| IBIS file generated by GenIBIS.pl Version 2.11
|   omap3530cbb
[IBIS ver]   4.1
[File name]   omap3530cbb.ibs
[File Rev]   1.0
[Date]   Wed Dec 9, 2009, 14:25:37
[Source]   Data created at Texas Instruments
[Notes]   1) Model checked with IBISCHK4 and contains...
   16 errors relating to DC endpoints. These errors can be waived
   and relate to special modelling of active feedback IOs.
   182 warnings relating to non-monotonic behavior, non-zero
   GND/POWER Clamp values and C_comp max/min values. These
   warnings can be waived.
[Disclaimer] Please be aware that in the absence of a written agreement,
   Texas Instruments (TI) assumes no liability for: 1) the
   accuracy of the IBIS models provided to your company, 2) the
   proper functioning of these IBIS models in your design or for
   any resulting applications, or, 3) infringement of patents,
   copyrights, or intellectual property rights resulting from
   your use of these IBIS models. TI provides IBIS models as a
   service to our customers and therefore reserves the right to
   limit distribution of the IBIS models.
[Copyright]   Property of Texas Instruments Incorporated. Unauthorised
   reproduction and/or distribution is strictly prohibited. This
   product is protected under copyright law and trade secret law
   as an unpublished work. Created 1999,(C) Copyright 1999-2001,
   Texas Instruments Incorporated., All Rights Reserved. These
   commodities are under the U.S. Government distribution license
   control.As such,they are not to be re-exported without the
   prior approval of the U.S. Department of Commerce.
|   Component omap3530cbb
[Component]   omap3530cbb
[Manufacturer]   Texas Instruments.
[Package Model] omap3530cbb
[Package]
|   typ   min   max
R_pkg   0.4048305   2.97780e-002   7.79883e-001
L_pkg   4.2681365E-009 -2.79127e-010  8.81540e-009
C_pkg   1.649116E-012  -6.89568e-013  3.98780e-012
[Pin]   signal_name   model_name
A4   sdrc_a0   Selector8
A6   sdrc_dqs0   Selector1
A7   sdrc_d5   Selector11
A9   sdrc_d7   Selector11
A10   sdrc_dqs2   Selector1
A11   sdrc_d21   Selector11
A16   sdrc_dm1   Selector8
A17   sdrc_dqs1   Selector1
A19   sdrc_d25   Selector11
A20   sdrc_dqs3   Selector1
A25   cam_d5   Selector1
AA3   mcspi2_clk   Selector1
AA4   mcspi1_somi   Selector15
AA8   uart1_tx   Selector1
AA9   uart1_rts   Selector1
AA12   jtag_rtck   Selector6
AA17   jtag_ntrst   Selector27
AA19   jtag_tdo   Selector6
AA25   uart2_tx   Selector23
AA27   dss_data15   Selector24
AA28   dss_data14   Selector24
AB1   mcspi1_cs2   Selector15
AB4   mcspi1_simo   Selector15
AB25   uart2_rts   Selector23
AB26   uart2_cts   Selector23
AB27   dss_data13   Selector24
AC3   mcspi1_cs1   Selector15
AC27   dss_data22   Selector24
AD1   mcbsp4_dr   Selector1
AD27   dss_data11   Selector24
AE1   mcbsp4_clkx   Selector1
AE3   mmc2_dat7   Selector1
AE5   mcbsp3_fsx   Selector1
AE7   etk_d10   Selector1
AE10   etk_ctl   Selector17
AE11   etk_d4   Selector1
AE14   sys_boot2   Selector19
AE17   sys_xtalin   Model79
AE21   sys_boot5   Selector19
AE25   sys_32k   Model94
AF3   mmc2_dat6   Selector1
AF6   mcbsp3_dx   Selector1
AF7   etk_d11   Selector1
AF9   etk_d8   Selector1
AF10   etk_clk   Selector17
AF14   i2c3_scl   Selector9
AF15   i2c2_scl   Selector9
AF18   sys_boot3   Selector19
AF19   sys_boot4   Selector19
AF22   sys_off_mode   Selector25
AF24   sys_nreswarm   Selector25
AF25   sys_clkreq   Selector25
AG4   mmc2_dat2   Selector17
AG9   etk_d9   Selector1
AG14   i2c3_sda   Selector9
AG18   gpio_114   Selector14
AG19   gpio_112   Selector30
AG22   dss_data0   Model23
AG24   dss_data4   Model23
AG25   sys_clkout1   Selector6
AH9   etk_d5   Selector1
AH14   etk_d7   Selector1
AH17   cam_d1   Selector4
AH19   gpio_113   Selector12
AH22   dss_data1   Model23
AA21   mcbsp1_fsr   Selector1
AB2   mcspi1_cs3   Selector17
AC1   mcbsp4_fsx   Selector1
AD2   mcbsp4_dx   Selector1
AD28   dss_data10   Selector24
AE6   mcbsp3_dr   Selector1
A23   cam_vs   Selector1
AA18   jtag_tms_tmsc   Selector31
AC2   mcspi1_cs0   Selector15
AE22   sys_clkout2   Selector1
AF4   mmc2_dat3   Selector17
AG17   cam_d0   Selector21
AH7   etk_d13   Selector1
AH23   dss_data3   Model23
AH25   sys_nrespwron   Model75
AD25   uart2_rx   Selector23
AD26   i2c4_scl   Selector22
AE15   i2c2_sda   Selector9
AH24   dss_data5   Model23
A21   sdrc_d29   Selector11
A24   cam_hs   Selector1
AA20   jtag_tdi   Model74
AB3   mcspi1_clk   Selector15
AB28   dss_data12   Selector24
AE4   mmc2_dat4   Selector1
AE26   i2c4_sda   Selector22
A14   sdrc_nclk   Selector13
AA11   jtag_emu0   Selector23
AF21   sys_boot6   Selector19
AF26   sys_nirq   Selector23
AG5   mmc2_cmd   Selector17
AG7   etk_d12   Selector1
AG8   etk_d14   Selector1
AG23   dss_data2   Model23
AH3   mmc2_dat5   Selector1
AH5   mmc2_dat0   Selector17
AH8   etk_d15   Selector1
AH12   etk_d2   Selector17
AH18   gpio_115   Selector32
AH26   sys_boot0   Selector19
A13   sdrc_clk   Selector1
AA10   jtag_emu1   Selector23
AA13   jtag_tck   Selector27
AC28   dss_data23   Selector24
AE2   mmc2_clk   Selector1
AE13   etk_d3   Selector17
AF5   mcbsp3_clkx   Selector1
AF11   etk_d0   Selector17
AF13   etk_d6   Selector1
AG12   etk_d1   Selector1
AG26   sys_boot1   Selector19
AH4   mmc2_dat1   Selector17
B3   sdrc_a2   Selector8
B4   sdrc_a1   Selector8
B6   sdrc_d2   Selector11
B7   sdrc_dm0   Selector8
B9   sdrc_d6   Selector11
B10   sdrc_d17   Selector11
B11   sdrc_dm2   Selector8
B13   sdrc_d22   Selector11
B14   sdrc_d9   Selector11
B16   sdrc_d11   Selector11
B17   sdrc_d14   Selector11
B19   sdrc_d26   Selector11
B20   sdrc_d27   Selector11
B21   sdrc_d30   Selector11
B23   cam_wen   Selector1
B24   cam_d2   Selector1
B25   cam_d10   Selector1
B26   cam_xclkb   Selector1
C1   sdrc_a8   Selector8
C2   sdrc_a7   Selector8
C3   sdrc_a6   Selector8
C4   sdrc_a4   Selector8
C5   sdrc_a3   Selector8
C6   sdrc_d1   Selector11
C8   sdrc_d3   Selector11
C9   sdrc_d4   Selector11
C11   sdrc_d18   Selector11
C12   sdrc_d20   Selector11
C14   sdrc_d8   Selector11
C15   sdrc_d10   Selector11
C17   sdrc_d13   Selector11
C18   sdrc_d24   Selector11
C20   sdrc_dm3   Selector8
C21   sdrc_d31   Selector11
C23   cam_fld   Selector1
C24   cam_d3   Selector1
C25   cam_xclka   Selector1
C26   cam_d11   Selector1
C27   cam_pclk   Selector1
D1   sdrc_a12   Selector8
D2   sdrc_a11   Selector8
D3   sdrc_a10   Selector8
D4   sdrc_a9   Selector8
D5   sdrc_a5   Selector8
D6   sdrc_d0   Selector11
D11   sdrc_d16   Selector11
D12   sdrc_d19   Selector11
D14   sdrc_d23   Selector11
D17   sdrc_d12   Selector11
D18   sdrc_d15   Selector11
D20   sdrc_d28   Selector11
D24   cam_d4   Selector1
D25   cam_strobe   Selector1
D26   dss_hsync   Selector2
D27   dss_vsync   Selector2
D28   dss_pclk   Selector2
E1   sdrc_a14   Selector8
E2   sdrc_a13   Selector8
E26   dss_data6   Selector10
E27   dss_acbias   Selector10
E28   dss_data20   Selector2
F3   gpmc_nadv_ale   Selector8
F4   gpmc_nwe   Selector13
F27   dss_data8   Selector10
F28   dss_data7   Selector10
G2   gpmc_noe   Selector13
G3   gpmc_nbe0_cle   Selector1
G4   gpmc_ncs0   Selector13
G25   dss_data16   Selector10
G26   dss_data9   Selector10
H1   gpmc_nwp   Selector1
H2   gpmc_d8   Selector17
H3   gpmc_ncs1   Selector17
H9   sdrc_ba0   Selector8
H10   sdrc_ba1   Selector8
H11   sdrc_ncs0   Selector13
H12   sdrc_ncs1   Selector13
H13   sdrc_ncas   Selector13
H14   sdrc_nras   Selector13
H15   sdrc_nwe   Selector13
H16   sdrc_cke0   Selector3
H17   sdrc_cke1   Selector3
H18   uart3_cts_rctx   Selector23
H19   uart3_rts_sd   Selector23
H20   uart3_rx_irrx   Selector23
H21   uart3_tx_irtx   Selector23
H25   dss_data19   Selector10
H26   dss_data18   Selector10
H27   dss_data17   Selector10
J8   gpmc_wait3   Selector17
J21   i2c1_sda   Selector5
J25   hdq_sio   Selector23
J26   dss_data21   Selector10
K1   gpmc_d0   Selector17
K2   gpmc_d9   Selector17
K3   gpmc_a10   Selector17
K4   gpmc_a4   Selector1
K8   gpmc_wait2   Selector17
K21   i2c1_scl   Selector5
K26   mcbsp1_fsx   Selector1
K27   cam_d8   Selector16
K28   cam_d6   Selector20
L1   gpmc_d1   Selector17
L2   gpmc_d2   Selector17
L3   gpmc_a9   Selector17
L4   gpmc_a3   Selector1
L8   gpmc_wait1   Selector17
L27   cam_d9   Selector18
L28   cam_d7   Selector29
M3   gpmc_a8   Selector17
M4   gpmc_a2   Selector1
M8   gpmc_wait0   Selector26
M21   mcbsp2_dx   Selector15
M27   mmc1_cmd   Selector28
N3   gpmc_a7   Selector17
N4   gpmc_a1   Selector1
N8   gpmc_ncs7   Selector17
N21   mcbsp2_clkx   Selector15
N25   mmc1_dat2   Selector28
N26   mmc1_dat1   Selector28
N27   mmc1_dat0   Selector28
N28   mmc1_clk   Selector28
P1   gpmc_d10   Selector17
P2   gpmc_d3   Selector17
P8   gpmc_ncs6   Selector17
P21   mcbsp2_fsx   Selector15
P26   mmc1_dat5   Selector7
P27   mmc1_dat4   Selector7
P28   mmc1_dat3   Selector28
R1   gpmc_d11   Selector17
R2   gpmc_d12   Selector17
R3   gpmc_a6   Selector17
R8   gpmc_ncs5   Selector17
R21   mcbsp2_dr   Selector15
R25   mmc1_dat7   Selector7
R27   mmc1_dat6   Selector7
R28   hsusb0_dir   Selector1
T1   gpmc_d4   Selector17
T2   gpmc_d13   Selector17
T3   gpmc_a5   Selector1
T4   gpmc_clk   Selector1
T8   gpmc_ncs4   Selector17
T21   mcbsp_clks   Selector1
T25   hsusb0_stp   Selector17
T26   hsusb0_nxt   Selector1
T27   hsusb0_data0   Selector1
T28   hsusb0_clk   Selector1
U3   gpmc_nbe1   Selector1
U8   gpmc_ncs3   Selector17
U21   mcbsp1_dr   Selector1
U25   hsusb0_data4   Selector1
U26   hsusb0_data3   Selector1
U27   hsusb0_data2   Selector1
U28   hsusb0_data1   Selector1
V1   gpmc_d5   Selector17
V2   gpmc_d6   Selector17
V3   mcspi2_cs1   Selector1
V8   gpmc_ncs2   Selector17
V21   mcbsp1_dx   Selector1
V26   hsusb0_data7   Selector1
V27   hsusb0_data6   Selector1
V28   hsusb0_data5   Selector1
W1   gpmc_d14   Selector17
W2   gpmc_d7   Selector17
W8   uart1_cts   Selector1
W21   mcbsp1_clkx   Selector1
Y1   gpmc_d15   Selector17
Y2   mcspi2_simo   Selector1
Y3   mcspi2_somi   Selector1
Y4   mcspi2_cs0   Selector17
Y8   uart1_rx   Selector1
Y21   mcbsp1_clkr   Selector1
| Device pads which are not required to be modeled. Included for completeness
|A1   No Connect   PASS
|A2   FeedThrough Pins   PWR
|A3   vss   GND
|A5   vdds_mem   PWR
|A8   vdds_mem   PWR
|A18   vdds_mem   PWR
|A27   FeedThrough Pins   PWR
|AA1   FeedThrough Pins   PWR
|AA2   FeedThrough Pins   PWR
|AA15   cap_vdd_d   GND
|AA16   vdds_dpll_per   PWR
|AC4   vdd_core   PWR
|AC25   vss   GND
|AC26   vss   GND
|AE9   vdd_core   PWR
|AE16   vdds   PWR
|AE19   vdd_core   PWR
|AE23   vdds   PWR
|AE24   vdd_core   PWR
|A28   FeedThrough Pins   PWR
|AF1   FeedThrough Pins   PWR
|AF2   FeedThrough Pins   PWR
|AF8   vdds   PWR
|AF12   vss   GND
|AF16   vdds   PWR
|AF20   vss   GND
|AF23   vdds   PWR
|AF27   FeedThrough Pins   PWR
|AG1   FeedThrough Pins   PWR
|AG2   vss   GND
|AG3   vss   GND
|AG10   FeedThrough Pins   PWR
|AG11   FeedThrough Pins   PWR
|AG16   vss   GND
|AG20   vdds   PWR
|AG21   vdds   PWR
|AG27   vdds   PWR
|AG28   FeedThrough Pins   PWR
|AH1   FeedThrough Pins   PWR
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[Model Selector] Selector1
Model4 1.8V-I/O-X-SLOW
Model5 1.8V-I/O-X-FAST
Model6 1.8V-INPUT-PD-X
Model7 1.8V-INPUT-PI-X
Model8 1.8V-INPUT-PU-X
| Model selector for model set 1,2,3
|   Usage O#1.8V#PD/PI/PU##BQ0232CS_7LM
[Model Selector] Selector2
Model1 1.8V-I/O-PD-X
Model2 1.8V-I/O-PI-X
Model3 1.8V-I/O-PU-X
| Model selector for model set 10,9
|   Usage O#1.8V#PD/PI/PU##BQ0268CS_7LM
[Model Selector] Selector3
Model10 1.8V-I/O-X-FAST
Model9 1.8V-I/O-X-SLOW
| Model selector for model set 11,12
|   Usage I#1.8V###CSI2PHY3LANE_7LM.8
[Model Selector] Selector4
Model11 1.8V-INPUT-X-X-LPRX Mode
Model12 1.8V-INPUT-X-X-GPI mode
| Model selector for model set 13,14
|   Usage IOOD#1.8V#PD/PI/PU##BQ0246S_7LM
[Model Selector] Selector5
Model13 1.8000V-I/O_OPEN_DRAIN-X-STANDARD
Model14 1.8000V-I/O_OPEN_DRAIN-X-LOWC
| Model selector for model set 15,16,17
|   Usage O#1.8V###BQ0253CS_7LM
[Model Selector] Selector6
Model15 1.8V-I/O-PD-X
Model16 1.8V-I/O-PI-X
Model17 1.8V-I/O-PU-X
| Model selector for model set 18,19,20
|   Usage IO#1.8V#PD/PI/PU##BQ0447S_7LM
[Model Selector] Selector7
Model18 1.8V-I/O-PD-X
Model19 1.8V-I/O-PI-X
Model20 1.8V-I/O-PU-X
| Model selector for model set 21,22
|   Usage O#1.8V#PD/PI/PU##OQ0163CS_7LM
[Model Selector] Selector8
Model21 1.8V-3-STATE-X-SLOW
Model22 1.8V-3-STATE-X-FAST
| Model selector for model set 13,14,27,28
|   Usage IO#1.8V#PD/PI/PU##BQ0246S_7LM
|   IOOD#1.8V#PD/PI/PU##BQ0246S_7LM
[Model Selector] Selector9
Model13 1.8000V-I/O_OPEN_DRAIN-X-STANDARD
Model14 1.8000V-I/O_OPEN_DRAIN-X-LOWC
Model27 1.8000V-I/O-X-X
Model28 1.8000V-I/O-X-HIGHC
| Model selector for model set 24,25,26
|   Usage O#1.8V#PD/PI/PU##BQ0230CS_7LM
[Model Selector] Selector10
Model24 1.8V-I/O-PD-X
Model25 1.8V-I/O-PI-X
Model26 1.8V-I/O-PU-X
| Model selector for model set 5,6,7,8
|   Usage IO#1.8V#PD/PI/PU#FAST#BQ0267CS_7LM
[Model Selector] Selector11
Model5 1.8V-I/O-X-FAST
Model6 1.8V-INPUT-PD-X
Model7 1.8V-INPUT-PI-X
Model8 1.8V-INPUT-PU-X
| Model selector for model set 29,30
|   Usage I#1.8V###CSI2PHY3LANE_7LM.4
[Model Selector] Selector12
Model29 1.8V-INPUT-X-X-LPRX Mode
Model30 1.8V-INPUT-X-X-GPI mode
| Model selector for model set 31,32
|   Usage O#1.8V#PD/PI/PU##OQ0164CS_7LM
[Model Selector] Selector13
Model31 1.8V-3-STATE-X-SLOW
Model32 1.8V-3-STATE-X-FAST
| Model selector for model set 33,34
|   Usage I#1.8V###CSI2PHY3LANE_7LM.5
[Model Selector] Selector14
Model33 1.8V-INPUT-X-X-LPRX Mode
Model34 1.8V-INPUT-X-X-GPI mode
| Model selector for model set 35,36,37,38,39,40,41,42,43,44,45,46
|   Usage O#1.8V#PD/PI/PU##BQOMAPPROGIOCSHYFBPB_7LM
[Model Selector] Selector15
Model35 1.8V-I/O-PD-DS00
Model36 1.8V-I/O-PD-DS11
Model37 1.8V-I/O-PD-DS10
Model38 1.8V-I/O-PD-DS01
Model39 1.8V-I/O-PI-DS11
Model40 1.8V-I/O-PI-DS10
Model41 1.8V-I/O-PI-DS01
Model42 1.8V-I/O-PI-DS00
Model43 1.8V-I/O-PU-DS00
Model44 1.8V-I/O-PU-DS11
Model45 1.8V-I/O-PU-DS10
Model46 1.8V-I/O-PU-DS01
| Model selector for model set 47,48,49
|   Usage I#1.8V#PD/PI/PU##CCPV2_7LM.3
[Model Selector] Selector16
Model47 1.8V-I/O-PD-X
Model48 1.8V-I/O-PI-X
Model49 1.8V-I/O-PU-X
| Model selector for model set 10,50,51,52,9
|   Usage IO#1.8V#PD/PI/PU##BQ0268CS_7LM
|   O#1.8V#PD/PU##BQ0268CS_7LM
[Model Selector] Selector17
Model10 1.8V-I/O-X-FAST
Model50 1.8V-INPUT-PD-X
Model51 1.8V-INPUT-PI-X
Model52 1.8V-INPUT-PU-X
Model9 1.8V-I/O-X-SLOW
| Model selector for model set 53,54,55
|   Usage I#1.8V#PD/PI/PU##CCPV2_7LM.4
[Model Selector] Selector18
Model53 1.8V-I/O-PD-X
Model54 1.8V-I/O-PI-X
Model55 1.8V-I/O-PU-X
| Model selector for model set 56,57,58
|   Usage IO#1.8V#PD/PI/PU##BQ0228CS_7LM
[Model Selector] Selector19
Model56 1.8V-I/O-PD-X
Model57 1.8V-I/O-PI-X
Model58 1.8V-I/O-PU-X
| Model selector for model set 59,60,61
|   Usage I#1.8V#PD/PI/PU##CCPV2_7LM.1
[Model Selector] Selector20
Model59 1.8V-I/O-PD-X
Model60 1.8V-I/O-PI-X
Model61 1.8V-I/O-PU-X
| Model selector for model set 62,63
|   Usage I#1.8V###CSI2PHY3LANE_7LM.7
[Model Selector] Selector21
Model62 1.8V-INPUT-X-X-LPRX Mode
Model63 1.8V-INPUT-X-X-GPI mode
| Model selector for model set 64,65,66,67
|   Usage IOOD#1.8V#PD/PI/PU##BQ0245S_7LM
|   O#1.8V#PD/PI/PU##BQ0245S_7LM
[Model Selector] Selector22
Model64 1.8000V-I/O_OPEN_DRAIN-X-STANDARD
Model65 1.8000V-I/O_OPEN_DRAIN-X-LOWC
Model66 1.8000V-I/O-X-X
Model67 1.8000V-I/O-X-HIGHC
| Model selector for model set 68,69,70
|   Usage IO#1.8V#PD/PI/PU##BQ0226CS_7LM
[Model Selector] Selector23
Model68 1.8V-I/O-PD-X
Model69 1.8V-I/O-PI-X
Model70 1.8V-I/O-PU-X
| Model selector for model set 71,72,73
|   Usage IO#1.8V#PD/PI/PU##SDI2_7LM
[Model Selector] Selector24
Model71 1.8V-I/O-PD-X
Model72 1.8V-I/O-PU-X
Model73 1.8V-I/O-PI-X
| Model selector for model set 76,77,78
|   Usage IO#1.8V#PD/PI/PU##BQ0234CS_7LM
[Model Selector] Selector25
Model76 1.8V-I/O-PD-X
Model77 1.8V-I/O-PI-X
Model78 1.8V-I/O-PU-X
| Model selector for model set 80,81,82
|   Usage I#1.8V#PD/PI/PU##IQ0101CS_7LM
[Model Selector] Selector26
Model80 1.8V-INPUT-PD-X
Model81 1.8V-INPUT-PI-X
Model82 1.8V-INPUT-PU-X
| Model selector for model set 83,84,85
|   Usage I#1.8V###IQ0120CS_7LM
[Model Selector] Selector27
Model83 1.8V-INPUT-PD-X
Model84 1.8V-INPUT-PU-X
Model85 1.8V-INPUT-PI-X
| Model selector for model set 86,87,88
|   Usage IO#1.8V#PD/PI/PU##BQ0247S_7LM
|   IO#1.8V3.0V#PD/PI/PU##BQ0247S_7LM
[Model Selector] Selector28
Model86 1.8000V-I/O-PD-X
Model87 1.8000V-I/O-PI-X
Model88 1.8000V-I/O-PU-X
| Model selector for model set 95,96,97
|   Usage I#1.8V#PD/PI/PU##CCPV2_7LM.2
[Model Selector] Selector29
Model95 1.8V-I/O-PD-X
Model96 1.8V-I/O-PI-X
Model97 1.8V-I/O-PU-X
| Model selector for model set 92,93
|   Usage I#1.8V###CSI2PHY3LANE_7LM.3
[Model Selector] Selector30
Model92 1.8V-INPUT-X-X-LPRX Mode
Model93 1.8V-INPUT-X-X-GPI mode
| Model selector for model set 89,90,91
|   Usage IO#1.8V###BQ0254CS_7LM
[Model Selector] Selector31
Model89 1.8V-I/O-PD-X
Model90 1.8V-I/O-PU-X
Model91 1.8V-I/O-PI-X
| Model selector for model set 98,99
|   Usage I#1.8V###CSI2PHY3LANE_7LM.6
[Model Selector] Selector32
Model98 1.8V-INPUT-X-X-LPRX Mode
Model99 1.8V-INPUT-X-X-GPI mode
| Package model definition
[Define Package Model]  omap3530cbb
[Manufacturer]   Texas Instruments.
[OEM]   Texas Instruments.
[Description]   omap3530cbb package model generated by GenIBIS.pl
[Number Of Pins]   289
[Pin Numbers]
A4   | 1 sdrc_a0   O
A6   | 2 sdrc_dqs0   IO
A7   | 3 sdrc_d5   IO
A9   | 4 sdrc_d7   IO
A10   | 5 sdrc_dqs2   IO
A11   | 6 sdrc_d21   IO
A16   | 7 sdrc_dm1   O
A17   | 8 sdrc_dqs1   IO
A19   | 9 sdrc_d25   IO
A20   | 10 sdrc_dqs3   IO
A25   | 11 cam_d5   IO
AA3   | 12 mcspi2_clk   IO
AA4   | 13 mcspi1_somi   IO
AA8   | 14 uart1_tx   IO
AA9   | 15 uart1_rts   IO
AA12   | 16 jtag_rtck   O
AA17   | 17 jtag_ntrst   I
AA19   | 18 jtag_tdo   O
AA25   | 19 uart2_tx   IO
AA27   | 20 dss_data15   IO
AA28   | 21 dss_data14   IO
AB1   | 22 mcspi1_cs2   IO
AB4   | 23 mcspi1_simo   IO
AB25   | 24 uart2_rts   IO
AB26   | 25 uart2_cts   IO
AB27   | 26 dss_data13   IO
AC3   | 27 mcspi1_cs1   O
AC27   | 28 dss_data22   O
AD1   | 29 mcbsp4_dr   IO
AD27   | 30 dss_data11   IO
AE1   | 31 mcbsp4_clkx   IO
AE3   | 32 mmc2_dat7   IO
AE5   | 33 mcbsp3_fsx   IO
AE7   | 34 etk_d10   O
AE10   | 35 etk_ctl   O
AE11   | 36 etk_d4   IO
AE14   | 37 sys_boot2   IO
AE17   | 38 sys_xtalin   I
AE21   | 39 sys_boot5   IO
AE25   | 40 sys_32k   I
AF3   | 41 mmc2_dat6   IO
AF6   | 42 mcbsp3_dx   IO
AF7   | 43 etk_d11   I
AF9   | 44 etk_d8   O
AF10   | 45 etk_clk   I
AF14   | 46 i2c3_scl   IO
AF15   | 47 i2c2_scl   IO
AF18   | 48 sys_boot3   IO
AF19   | 49 sys_boot4   IO
AF22   | 50 sys_off_mode   IO
AF24   | 51 sys_nreswarm   IO
AF25   | 52 sys_clkreq   IO
AG4   | 53 mmc2_dat2   IO
AG9   | 54 etk_d9   O
AG14   | 55 i2c3_sda   IO
AG18   | 56 gpio_114   I
AG19   | 57 gpio_112   I
AG22   | 58 dss_data0   IO
AG24   | 59 dss_data4   IO
AG25   | 60 sys_clkout1   IO
AH9   | 61 etk_d5   IO
AH14   | 62 etk_d7   IO
AH17   | 63 cam_d1   I
AH19   | 64 gpio_113   I
AH22   | 65 dss_data1   IO
AA21   | 66 mcbsp1_fsr   IO
AB2   | 67 mcspi1_cs3   IO
AC1   | 68 mcbsp4_fsx   IO
AD2   | 69 mcbsp4_dx   IO
AD28   | 70 dss_data10   IO
AE6   | 71 mcbsp3_dr   IO
A23   | 72 cam_vs   IO
AA18   | 73 jtag_tms_tmsc   IO
AC2   | 74 mcspi1_cs0   IO
AE22   | 75 sys_clkout2   IO
AF4   | 76 mmc2_dat3   IO
AG17   | 77 cam_d0   I
AH7   | 78 etk_d13   O
AH23   | 79 dss_data3   IO
AH25   | 80 sys_nrespwron   I
AD25   | 81 uart2_rx   IO
AD26   | 82 i2c4_scl   O
AE15   | 83 i2c2_sda   IO
AH24   | 84 dss_data5   IO
A21   | 85 sdrc_d29   IO
A24   | 86 cam_hs   IO
AA20   | 87 jtag_tdi   I
AB3   | 88 mcspi1_clk   IO
AB28   | 89 dss_data12   IO
AE4   | 90 mmc2_dat4   IO
AE26   | 91 i2c4_sda   O
A14   | 92 sdrc_nclk   O
AA11   | 93 jtag_emu0   IO
AF21   | 94 sys_boot6   IO
AF26   | 95 sys_nirq   IO
AG5   | 96 mmc2_cmd   IO
AG7   | 97 etk_d12   O
AG8   | 98 etk_d14   IO
AG23   | 99 dss_data2   IO
AH3   | 100 mmc2_dat5   IO
AH5   | 101 mmc2_dat0   IO
AH8   | 102 etk_d15   IO
AH12   | 103 etk_d2   IO
AH18   | 104 gpio_115   I
AH26   | 105 sys_boot0   IO
A13   | 106 sdrc_clk   IO
AA10   | 107 jtag_emu1   IO
AA13   | 108 jtag_tck   I
AC28   | 109 dss_data23   O
AE2   | 110 mmc2_clk   IO
AE13   | 111 etk_d3   IO
AF5   | 112 mcbsp3_clkx   IO
AF11   | 113 etk_d0   IO
AF13   | 114 etk_d6   IO
AG12   | 115 etk_d1   IO
AG26   | 116 sys_boot1   IO
AH4   | 117 mmc2_dat1   IO
B3   | 118 sdrc_a2   O
B4   | 119 sdrc_a1   O
B6   | 120 sdrc_d2   IO
B7   | 121 sdrc_dm0   O
B9   | 122 sdrc_d6   IO
B10   | 123 sdrc_d17   IO
B11   | 124 sdrc_dm2   O
B13   | 125 sdrc_d22   IO
B14   | 126 sdrc_d9   IO
B16   | 127 sdrc_d11   IO
B17   | 128 sdrc_d14   IO
B19   | 129 sdrc_d26   IO
B20   | 130 sdrc_d27   IO
B21   | 131 sdrc_d30   IO
B23   | 132 cam_wen   IO
B24   | 133 cam_d2   IO
B25   | 134 cam_d10   IO
B26   | 135 cam_xclkb   IO
C1   | 136 sdrc_a8   O
C2   | 137 sdrc_a7   O
C3   | 138 sdrc_a6   O
C4   | 139 sdrc_a4   O
C5   | 140 sdrc_a3   O
C6   | 141 sdrc_d1   IO
C8   | 142 sdrc_d3   IO
C9   | 143 sdrc_d4   IO
C11   | 144 sdrc_d18   IO
C12   | 145 sdrc_d20   IO
C14   | 146 sdrc_d8   IO
C15   | 147 sdrc_d10   IO
C17   | 148 sdrc_d13   IO
C18   | 149 sdrc_d24   IO
C20   | 150 sdrc_dm3   O
C21   | 151 sdrc_d31   IO
C23   | 152 cam_fld   IO
C24   | 153 cam_d3   IO
C25   | 154 cam_xclka   IO
C26   | 155 cam_d11   IO
C27   | 156 cam_pclk   IO
D1   | 157 sdrc_a12   O
D2   | 158 sdrc_a11   O
D3   | 159 sdrc_a10   O
D4   | 160 sdrc_a9   O
D5   | 161 sdrc_a5   O
D6   | 162 sdrc_d0   IO
D11   | 163 sdrc_d16   IO
D12   | 164 sdrc_d19   IO
D14   | 165 sdrc_d23   IO
D17   | 166 sdrc_d12   IO
D18   | 167 sdrc_d15   IO
D20   | 168 sdrc_d28   IO
D24   | 169 cam_d4   IO
D25   | 170 cam_strobe   IO
D26   | 171 dss_hsync   IO
D27   | 172 dss_vsync   IO
D28   | 173 dss_pclk   IO
E1   | 174 sdrc_a14   O
E2   | 175 sdrc_a13   O
E26   | 176 dss_data6   IO
E27   | 177 dss_acbias   IO
E28   | 178 dss_data20   O
F3   | 179 gpmc_nadv_ale   O
F4   | 180 gpmc_nwe   O
F27   | 181 dss_data8   IO
F28   | 182 dss_data7   IO
G2   | 183 gpmc_noe   O
G3   | 184 gpmc_nbe0_cle   IO
G4   | 185 gpmc_ncs0   O
G25   | 186 dss_data16   IO
G26   | 187 dss_data9   IO
H1   | 188 gpmc_nwp   IO
H2   | 189 gpmc_d8   IO
H3   | 190 gpmc_ncs1   IO
H9   | 191 sdrc_ba0   O
H10   | 192 sdrc_ba1   O
H11   | 193 sdrc_ncs0   O
H12   | 194 sdrc_ncs1   O
H13   | 195 sdrc_ncas   O
H14   | 196 sdrc_nras   O
H15   | 197 sdrc_nwe   O
H16   | 198 sdrc_cke0   O
H17   | 199 sdrc_cke1   O
H18   | 200 uart3_cts_rctx   IO
H19   | 201 uart3_rts_sd   IO
H20   | 202 uart3_rx_irrx   IO
H21   | 203 uart3_tx_irtx   IO
H25   | 204 dss_data19   IO
H26   | 205 dss_data18   IO
H27   | 206 dss_data17   IO
J8   | 207 gpmc_wait3   IO
J21   | 208 i2c1_sda   IOOD
J25   | 209 hdq_sio   IO
J26   | 210 dss_data21   O
K1   | 211 gpmc_d0   IO
K2   | 212 gpmc_d9   IO
K3   | 213 gpmc_a10   IO
K4   | 214 gpmc_a4   IO
K8   | 215 gpmc_wait2   IO
K21   | 216 i2c1_scl   IOOD
K26   | 217 mcbsp1_fsx   IO
K27   | 218 cam_d8   I
K28   | 219 cam_d6   I
L1   | 220 gpmc_d1   IO
L2   | 221 gpmc_d2   IO
L3   | 222 gpmc_a9   IO
L4   | 223 gpmc_a3   IO
L8   | 224 gpmc_wait1   IO
L27   | 225 cam_d9   I
L28   | 226 cam_d7   I
M3   | 227 gpmc_a8   IO
M4   | 228 gpmc_a2   IO
M8   | 229 gpmc_wait0   I
M21   | 230 mcbsp2_dx   IO
M27   | 231 mmc1_cmd   IO
N3   | 232 gpmc_a7   IO
N4   | 233 gpmc_a1   IO
N8   | 234 gpmc_ncs7   IO
N21   | 235 mcbsp2_clkx   IO
N25   | 236 mmc1_dat2   IO
N26   | 237 mmc1_dat1   IO
N27   | 238 mmc1_dat0   IO
N28   | 239 mmc1_clk   IO
P1   | 240 gpmc_d10   IO
P2   | 241 gpmc_d3   IO
P8   | 242 gpmc_ncs6   IO
P21   | 243 mcbsp2_fsx   IO
P26   | 244 mmc1_dat5   IO
P27   | 245 mmc1_dat4   IO
P28   | 246 mmc1_dat3   IO
R1   | 247 gpmc_d11   IO
R2   | 248 gpmc_d12   IO
R3   | 249 gpmc_a6   IO
R8   | 250 gpmc_ncs5   IO
R21   | 251 mcbsp2_dr   IO
R25   | 252 mmc1_dat7   IO
R27   | 253 mmc1_dat6   IO
R28   | 254 hsusb0_dir   IO
T1   | 255 gpmc_d4   IO
T2   | 256 gpmc_d13   IO
T3   | 257 gpmc_a5   IO
T4   | 258 gpmc_clk   IO
T8   | 259 gpmc_ncs4   IO
T21   | 260 mcbsp_clks   I
T25   | 261 hsusb0_stp   IO
T26   | 262 hsusb0_nxt   IO
T27   | 263 hsusb0_data0   IO
T28   | 264 hsusb0_clk   IO
U3   | 265 gpmc_nbe1   IO
U8   | 266 gpmc_ncs3   IO
U21   | 267 mcbsp1_dr   IO
U25   | 268 hsusb0_data4   IO
U26   | 269 hsusb0_data3   IO
U27   | 270 hsusb0_data2   IO
U28   | 271 hsusb0_data1   IO
V1   | 272 gpmc_d5   IO
V2   | 273 gpmc_d6   IO
V3   | 274 mcspi2_cs1   IO
V8   | 275 gpmc_ncs2   IO
V21   | 276 mcbsp1_dx   IO
V26   | 277 hsusb0_data7   IO
V27   | 278 hsusb0_data6   IO
V28   | 279 hsusb0_data5   IO
W1   | 280 gpmc_d14   IO
W2   | 281 gpmc_d7   IO
W8   | 282 uart1_cts   O
W21   | 283 mcbsp1_clkx   IO
Y1   | 284 gpmc_d15   IO
Y2   | 285 mcspi2_simo   IO
Y3   | 286 mcspi2_somi   IO
Y4   | 287 mcspi2_cs0   IO
Y8   | 288 uart1_rx   IO
Y21   | 289 mcbsp1_clkr   IO
[Model Data]
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[End Model Data]
[End Package Model]
| Models and submodels in the file (99): Model1 (I/O), Model2 (I/O), Model3 (I/O), Model4 (I/O), Model5 (I/O), Model6 (Input), Model7 (Input), Model8 (Input), Model9 (I/O), Model10 (I/O), Model11 (Input), Model12 (Input), Model13 (I/O_open_drain), Model14 (I/O_open_drain), Model15 (I/O), Model16 (I/O), Model17 (I/O), Model18 (I/O), Model19 (I/O), Model20 (I/O), Model21 (3-state), Model22 (3-state), Model23 (I/O), Model24 (I/O), Model25 (I/O), Model26 (I/O), Model27 (I/O), Model28 (I/O), Model29 (Input), Model30 (Input), Model31 (3-state), Model32 (3-state), Model33 (Input), Model34 (Input), Model35 (I/O), Model36 (I/O), Model37 (I/O), Model38 (I/O), Model39 (I/O), Model40 (I/O), Model41 (I/O), Model42 (I/O), Model43 (I/O), Model44 (I/O), Model45 (I/O), Model46 (I/O), Model47 (I/O), Model48 (I/O), Model49 (I/O), Model50 (Input), Model51 (Input), Model52 (Input), Model53 (I/O), Model54 (I/O), Model55 (I/O), Model56 (I/O), Model57 (I/O), Model58 (I/O), Model59 (I/O), Model60 (I/O), Model61 (I/O), Model62 (Input), Model63 (Input), Model64 (I/O_open_drain), Model65 (I/O_open_drain), Model66 (I/O), Model67 (I/O), Model68 (I/O), Model69 (I/O), Model70 (I/O), Model71 (I/O), Model72 (I/O), Model73 (I/O), Model74 (Input), Model75 (Input), Model76 (I/O), Model77 (I/O), Model78 (I/O), Model79 (Input), Model80 (Input)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
